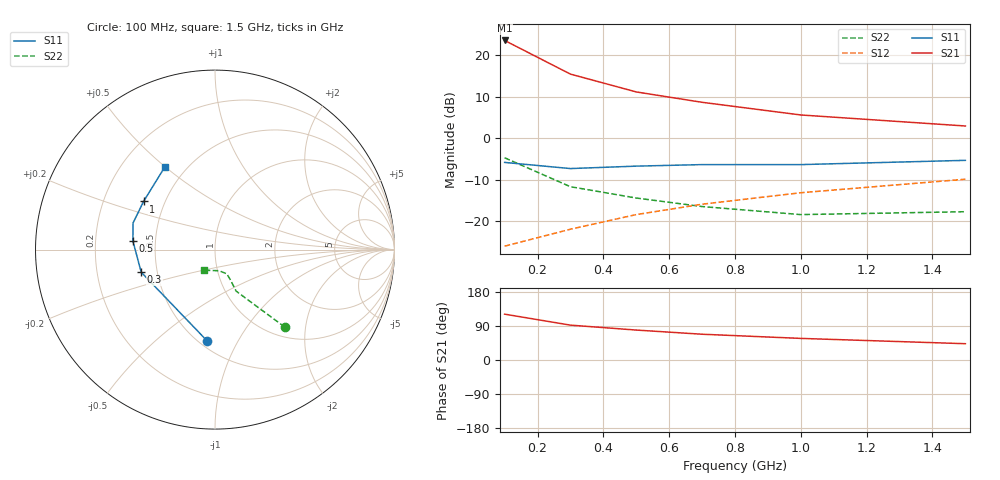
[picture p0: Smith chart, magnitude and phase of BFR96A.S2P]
! SCCS file tdata/motorola: @(#)get -r1.1 /eesof/src/tdata/motorola/s.bfr96a.s2p # Version date: 10/22/90
!  BFR96A.S2P
!  BFR96
!  VCE=5V; IC=10mA
#  GHZ S MA R 50
!  S-PARAMETER DATA
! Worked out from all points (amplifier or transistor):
!   6 points, 100 MHz to 1.5 GHz, reference 50 ohm
!   highest |S21| = 23.5 dB at 100 MHz (marker M1)
!   |S21| within 3 dB of that: start of sweep to 174 MHz
!   unconditionally stable (mu >= 1): 448.8 MHz to end of sweep
!   at 300 MHz: K = 0.93, MSG = 18.7 dB, |S12| = -21.9 dB
!   at 700 MHz: K = 1.03, MAG = 11.3 dB, |S12| = -15.9 dB
!   at 1.5 GHz: K = 1.01, MAG = 5.8 dB, |S12| = -9.9 dB
!   S11 on the Smith chart (normalised r, x): 100 MHz: 0.55, -0.75; 300 MHz: 0.41, -0.13; 500 MHz: 0.37, +0.05; 1 GHz: 0.38, +0.26; 1.5 GHz: 0.38, +0.50
0.1  0.51 -95.0  15 121.0  0.05 54.0  0.58 -48.0
0.3  0.43 -163.0  5.9 92.0  0.08 58.0  0.26 -63.0
0.5  0.46 174.0  3.6 79.0  0.12 63.0  0.19 -63.0
0.7  0.48 162.0  2.7 68.0  0.16 63.0  0.15 -64.0
1  0.48 146.0  1.9 57.0  0.22 63.0  0.12 -79.0
1.5  0.54 121.0  1.4 43.0  0.32 58.0  0.13 -118.0
